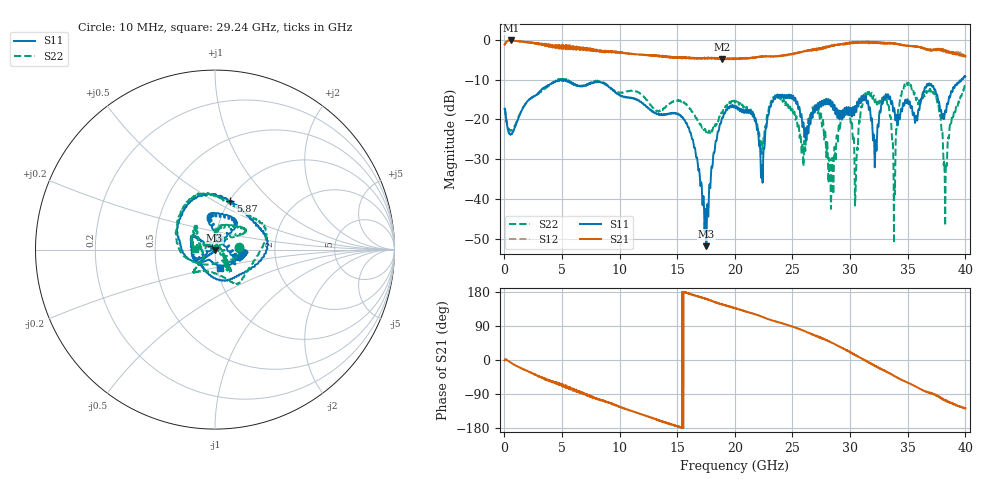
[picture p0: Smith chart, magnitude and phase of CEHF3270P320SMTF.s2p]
!Agilent Technologies,N5224A,MY51441447,A.10.00.00
!Agilent N5224A: A.10.00.00
!Date: Wednesday, January 15, 2020 17:58:42
!Correction: S11(Full 2 Port(1,2))
!S21(Full 2 Port(1,2))
!S12(Full 2 Port(1,2))
!S22(Full 2 Port(1,2))
!S2P File: Measurements: S11, S21, S12, S22:
# Hz S  dB  R 50
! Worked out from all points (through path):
!   4001 points, 10 MHz to 40.01 GHz, reference 50 ohm
!   highest |S21| = -0.21 dB at 560 MHz (marker M1); lowest = -4.9 dB at 18.86 GHz (marker M2)
!   group delay of S21, straight-line fit = 32.3 ps
!   lowest |S11| = -51.7 dB at 17.52 GHz (marker M3), VSWR 1.01, Z = 49.8 - j0.145 ohm
!   |S11| at or under -10 dB: start of sweep to 5.015 GHz; 5.024 GHz to 39.67 GHz (34.65 GHz wide, 155 % of centre)
!   |S22| runs from -51.0 to -9.7 dB; largest |S21 - S12| = 0.079
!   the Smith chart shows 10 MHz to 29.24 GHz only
!   S11 on the Smith chart (normalised r, x): 10 MHz: 1.31, +0.02; 5.87 GHz: 1.01, +0.59; 29.24 GHz: 1.03, -0.21
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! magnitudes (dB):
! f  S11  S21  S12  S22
! 10 MHz  -17.3  -1.2  -1.3  -17.3
! 560 MHz  -23.6  -0.2  -0.2  -22.8
! 5.87 GHz  -11.0  -1.9  -2.3  -10.8
! 6.68 GHz  -11.6  -2.4  -2.2  -11.7
! 13.35 GHz  -18.7  -4.1  -4.2  -18.0
! 15.84 GHz  -21.2  -4.5  -4.7  -16.5
! 17.52 GHz  -51.7  -4.5  -4.6  -23.0
! 18.86 GHz  -19.8  -4.9  -4.8  -18.2
! 20.01 GHz  -16.7  -4.8  -4.8  -15.8
! 22.38 GHz  -34.1  -4.2  -4.2  -27.5
! 23.56 GHz  -14.1  -4.2  -4.2  -14.4
! 26.68 GHz  -18.6  -2.7  -2.6  -18.2
! 28.39 GHz  -16.7  -1.5  -1.6  -34.4
! 29.24 GHz  -19.6  -1.2  -1.2  -19.3
! 30.5 GHz  -17.6  -0.7  -0.7  -35.3
! 31.32 GHz  -14.6  -0.6  -0.7  -13.4
! 33.35 GHz  -14.7  -0.9  -0.8  -16.4
! 33.81 GHz  -17.2  -1.0  -1.0  -51.0
! 34.7 GHz  -16.5  -1.5  -1.5  -11.5
! 37.14 GHz  -11.7  -2.7  -2.5  -12.7
! 38.26 GHz  -17.7  -2.7  -2.9  -45.1
! 40.01 GHz  -9.3  -4.1  -4.3  -11.4
